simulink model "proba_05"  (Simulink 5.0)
settings: Solver=ode45  SolverMode=SingleTasking  StartTime=0.0  StopTime=5.0  MaxStep=0.01  RelTol=1e-3  AbsTol=1e-6

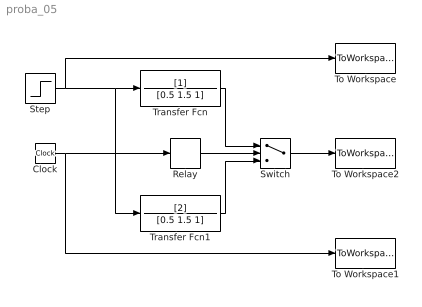
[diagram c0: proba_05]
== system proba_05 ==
  Clock : Clock
  Relay : Relay  OnSwitchValue=3  OffSwitchValue=3  OnOutputValue=-1  OffOutputValue=1
  Step : Step  Time=0  SampleTime=0
  Switch : Switch
  To Workspace : ToWorkspace  VariableName=ut  SampleTime=-1  SaveFormat=Array
  To Workspace1 : ToWorkspace  VariableName=u  SampleTime=-1  SaveFormat=Array
  To Workspace2 : ToWorkspace  VariableName=yt  SampleTime=-1  SaveFormat=Array
  Transfer Fcn : TransferFcn  Denominator=[0.5 1.5 1]
  Transfer Fcn1 : TransferFcn  Numerator=[2]  Denominator=[0.5 1.5 1]
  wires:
  Relay/1 -> Switch/2
  Transfer Fcn1/1 -> Switch/3
  Transfer Fcn/1 -> Switch/1
  Step/1 -> Transfer Fcn/1, Transfer Fcn1/1, To Workspace/1
  Clock/1 -> Relay/1, To Workspace1/1
  Switch/1 -> To Workspace2/1
